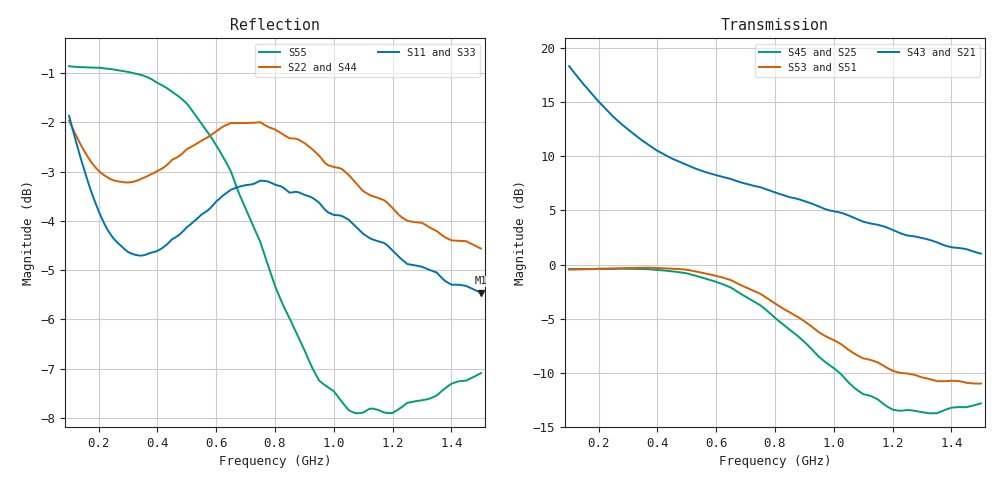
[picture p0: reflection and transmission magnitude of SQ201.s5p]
!  POLYFET RF DEVICES
!  S PARAMETERS FOR
!  SQ201 (Each Side)
!  VDS=28, IDQ=200MA
! S2A1Die, AP pkg, VDS=28VDC, IDQ=200ma, Vgsth=3.17Vdc
! Date: Thu Sep 24 14:28:25 1998
!AWR Design Environment (2053) Wed Feb 04 15:57:14 2004
!freq-unit  param-type  data-format  keyword  impedance-ohms
# MHz  S  MA  R  50
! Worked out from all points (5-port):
!   141 points, 100 MHz to 1.5 GHz, reference 50 ohm
!   strongest paths, dB at 100 MHz, 450 MHz, 800 MHz, 1.15 GHz, 1.5 GHz:
!     S43: 18.3, 9.8, 6.7, 3.7, 1.0
!     S21: 18.3, 9.8, 6.7, 3.7, 1.0
!     S53: -0.5, -0.4, -3.6, -9.0, -11.0
!     S51: -0.5, -0.4, -3.6, -9.0, -11.0
!     S45: -0.4, -0.6, -4.9, -12.5, -12.8
!     S25: -0.4, -0.6, -4.9, -12.5, -12.8
!   lowest |S11| = -5.5 dB at 1.5 GHz (marker M1), VSWR 3.29, Z = 15.2 + j0.907 ohm
!   |S11| at or under -10 dB: nowhere
